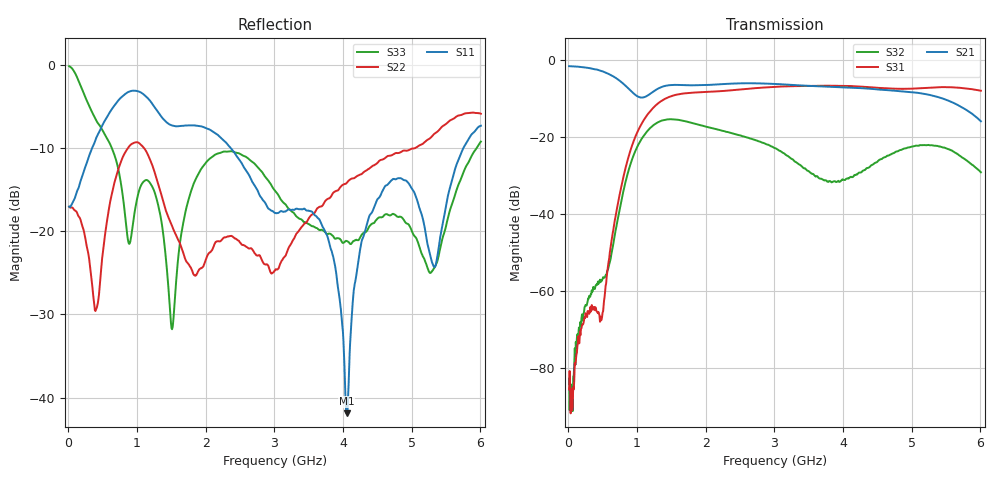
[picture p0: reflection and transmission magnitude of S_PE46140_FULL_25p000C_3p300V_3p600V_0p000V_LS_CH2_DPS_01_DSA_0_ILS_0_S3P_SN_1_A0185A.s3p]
! Device ID: PE46140_FULL
! File Path: z:\PE46140\MajorStates\25p000C\3p300\LS_CH2_DPS_01_DSA_0_ILS_0\PE46140_FULL_25p000C_3p300V_3p600V_0p000V_LS_CH2_DPS_01_DSA_0_ILS_0_S3P_SN_1_A0185A.s3p
! Serial: 1
! Lot: A0185A
! Temp: 25.000C
! VDD: 3.300
! VSS: 0.000
! Control_Hi: 3.600
! Control_Lo: 0.000
! Logic State: LS_CH2_DPS_01_DSA_0_ILS_0
! Port 1: RFIN
! Port 2: RFOUT1
! Port 3: RFOUT2
! ThroughPath:1-3
! IDD: 0.000314715
! ISS: -1.295e-007
! Comment:
#  Hz  S  RI  R  50
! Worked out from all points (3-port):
!   801 points, 10 MHz to 6.01 GHz, reference 50 ohm
!   strongest paths, dB at 10 MHz, 1.51 GHz, 3.01 GHz, 4.51 GHz, 6.01 GHz:
!     S21: -1.5, -6.4, -6.1, -7.6, -15.8
!     S31: -85.7, -9.2, -6.9, -7.1, -7.9
!     S32: -82.8, -15.3, -22.9, -26.2, -29.1
!   lowest |S11| = -41.9 dB at 4.053 GHz (marker M1), VSWR 1.02, Z = 49.3 + j0.37 ohm
!   |S11| at or under -10 dB: start of sweep to 346.1 MHz; 2.363 GHz to 5.756 GHz (3.393 GHz wide, 83.6 % of centre)
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1e7  0.1401 -0.0109  0.8421 -0.0244  2.13e-05 -4.16e-06
     0.8418 -0.0242  0.1399 -0.00674  -2.88e-05 2.14e-05
     5.82e-06 5.18e-05  2.98e-05 -6.58e-05  0.9747 -0.093
3.475e8  -0.00834 -0.3171  0.4735 -0.6216  -0.000453 -0.000354
         0.4732 -0.62  -0.00475 -0.0467  -0.00015 0.00099
         -0.000479 -0.000343  -0.000204 0.00095  -0.4457 -0.258
1.1725e9  -0.5665 0.2485  -0.1971 -0.2982  -0.2059 0.0271
          -0.1972 -0.2988  0.1996 -0.195  0.0327 0.1226
          -0.2062 0.0269  0.0326 0.1225  0.099 0.1723
1.51e9  -0.3476 0.255  -0.4476 -0.1718  0.0854 0.3345
        -0.4476 -0.1722  0.0348 -0.1015  0.1094 -0.1321
        0.0854 0.3349  0.1095 -0.1321  0.0136 0.0219
1.99e9  -0.1866 0.3736  -0.4099 0.2448  0.3695 -0.1162
        -0.4103 0.2448  0.0606 -0.024  -0.1385 0.00631
        0.3699 -0.116  -0.1384 0.00611  0.1482 0.2059
3.01e9  0.0178 0.1271  0.4113 0.273  -0.4017 -0.2107
        0.4111 0.274  -0.058 -0.00112  0.0625 -0.0353
        -0.402 -0.2109  0.0627 -0.0354  0.1549 -0.0811
3.76e9  0.0171 0.0943  0.2807 -0.3597  -0.2383 0.4042
        0.2814 -0.3593  0.0763 0.1341  -0.016 0.0219
        -0.2386 0.4043  -0.0159 0.0222  0.0841 -0.0474
4.0525e9  -0.00712 0.00376  0.0295 -0.4435  0.0185 0.4658
          0.0301 -0.4438  0.1432 0.1313  0.0256 0.013
          0.019 0.4658  0.0258 0.0129  0.0765 -0.0417
4.4875e9  -0.1302 -0.0766  -0.3178 -0.2748  0.3336 0.2893
          -0.3179 -0.2756  0.2411 0.0788  -0.00559 -0.0468
          0.3338 0.289  -0.0056 -0.0467  0.102 -0.057
6.01e9  -0.2944 -0.3128  0.1533 0.0485  -0.1993 -0.349
        0.1538 0.0486  0.2471 -0.4429  0.0298 -0.0186
        -0.2004 -0.35  0.0296 -0.0187  0.3154 0.1398
